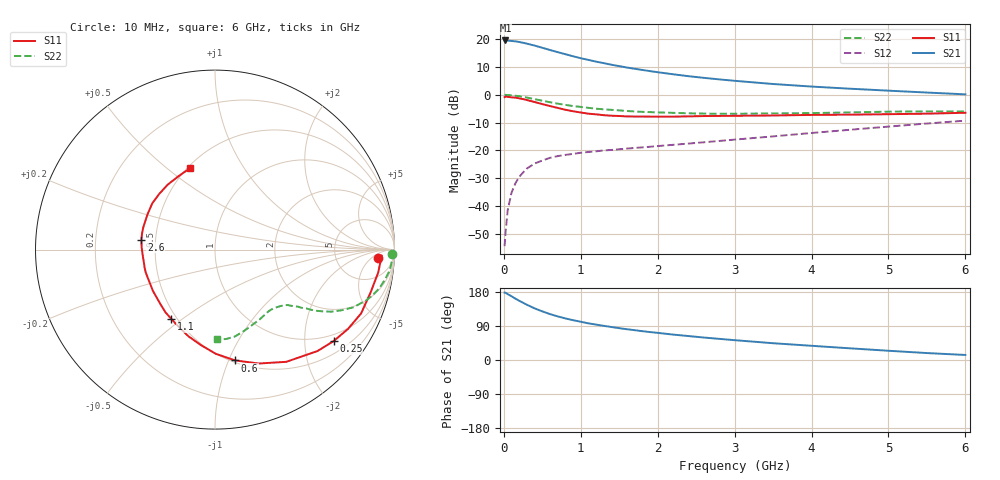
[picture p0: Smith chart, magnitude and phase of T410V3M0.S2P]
! Infineon Technologies  Discrete & RF Semiconductors
! BFR182T
! Si NPN RF Bipolar Junction Transistor in SC75
! VCE = 10 V  IC = 3 mA
! Common Emitter S-Parameters:  October  1999
# GHz  S  MA  R  50
!  f  S11  S21  S12  S22
! GHz  MAG  ANG  MAG  ANG  MAG  ANG  MAG  ANG
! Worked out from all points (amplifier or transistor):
!   36 points, 10 MHz to 6 GHz, reference 50 ohm
!   highest |S21| = 19.5 dB at 20 MHz (marker M1)
!   |S21| within 3 dB of that: start of sweep to 546.3 MHz
!   unconditionally stable (mu >= 1): 1.841 GHz to 4.363 GHz
!   at 250 MHz: K = 0.18, MSG = 23.3 dB, |S12| = -27.9 dB
!   at 1.4 GHz: K = 0.86, MSG = 15.3 dB, |S12| = -19.8 dB
!   at 6 GHz: K = 0.85, MSG = 4.7 dB, |S12| = -9.3 dB
!   S11 on the Smith chart (normalised r, x): 10 MHz: 17, -8; 250 MHz: 0.81, -2.72; 600 MHz: 0.52, -1.05; 1.1 GHz: 0.47, -0.46; 2.6 GHz: 0.42, +0.06; 6 GHz: 0.52, +0.61
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0.01  0.9086 -2.8  9.414 177.7  0.0019 71.6  0.9846 -1.4
0.02  0.9297 -2.0  9.463 177.6  0.0031 94.9  0.9972 -1.4
0.05  0.9183 -8.0  9.406 173.8  0.0084 89.1  0.9883 -3.5
0.1  0.8992 -15.4  9.257 168.2  0.0174 83.3  0.9797 -6.9
0.15  0.8884 -23.6  9.122 162.0  0.0256 77.2  0.961 -10.1
0.2  0.8629 -30.8  8.892 156.3  0.0334 75.1  0.9416 -13.1
0.25  0.8348 -37.6  8.601 151.0  0.0401 70.5  0.9164 -15.9
0.3  0.8035 -44.7  8.288 145.8  0.0473 66.9  0.8909 -18.4
0.4  0.7406 -57.6  7.653 136.2  0.0581 61.2  0.8344 -22.7
0.5  0.6798 -69.0  6.994 128.3  0.0658 57.0  0.7822 -25.6
0.6  0.6272 -79.8  6.373 121.1  0.0735 53.7  0.7344 -28.1
0.8  0.5377 -98.4  5.359 109.7  0.0831 49.5  0.6576 -31.2
0.9  0.5056 -106.9  4.915 105.1  0.0866 48.5  0.6268 -32.2
1.1  0.457 -122.1  4.23 96.7  0.0937 47.0  0.5815 -33.9
1.3  0.4293 -135.3  3.699 90.1  0.0999 47.0  0.5469 -35.3
1.6  0.4082 -152.5  3.086 81.2  0.1079 47.6  0.5109 -37.2
2.2  0.4043 -176.1  2.336 67.1  0.126 51.2  0.473 -42.5
2.6  0.4142 172.2  2.014 59.3  0.14 53.5  0.4585 -46.7
3.5  0.4242 152.5  1.561 44.3  0.1787 56.9  0.4616 -57.3
4.5  0.439 135.3  1.285 30.8  0.235 57.3  0.4817 -70.5
5.5  0.4572 116.1  1.096 18.3  0.3042 54.7  0.502 -83.0
6  0.4747 106.9  1.017 13.3  0.3427 52.1  0.5006 -88.5
